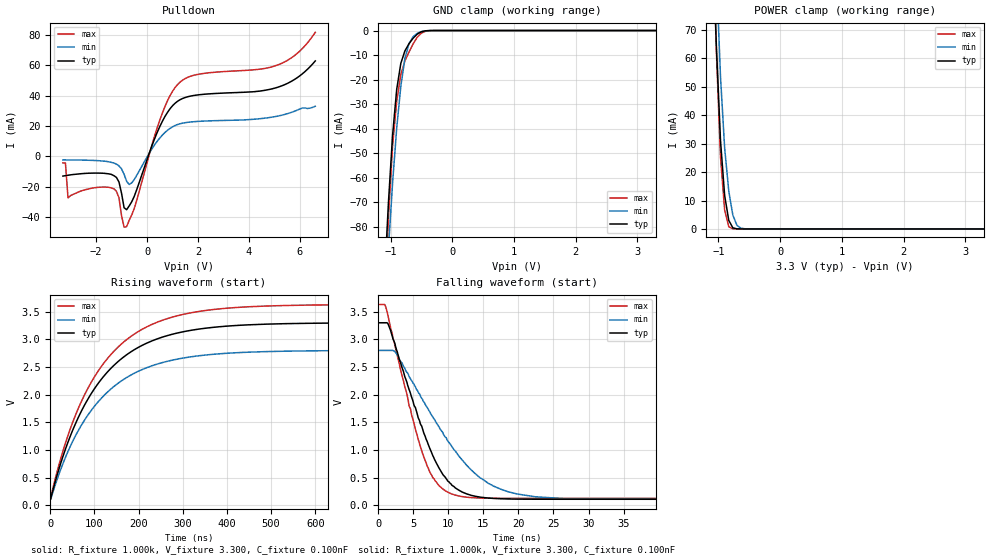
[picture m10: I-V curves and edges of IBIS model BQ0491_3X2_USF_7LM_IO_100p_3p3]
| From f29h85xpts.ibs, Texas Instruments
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|   Model BQ0491_3X2_USF_7LM_IO_100p_3p3
[Model]   BQ0491_3X2_USF_7LM_IO_100p_3p3
Model_type   I/O_open_drain
Polarity   Non-Inverting
Enable   Active-Low
Vinl =   0.800V
Vinh =   2.000V
Vmeas =  1.650V
Cref =   0.100nF
Rref =   1.000k
Vref =   3.300V
|   typ   min   max
C_comp   1.084pF   1.003pF   1.123pF
[Model Spec]
Vinh   2.000V   2.000V   2.000V
Vinl   0.800V   0.800V   0.800V
[Temperature Range]   25   155   -40
[Voltage Range]   3.300V   2.800V   3.630V
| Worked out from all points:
|   slope of the pulldown table from 0 to 0.495 V, typ, clamps not added: 22.9 ohm
|   GND clamp passes 1 mA (typ) near -0.53 V on its own axis
|   POWER clamp passes 1 mA (typ) near -0.78 V on its own axis
|   rising waveform, R_fixture 1.000k, V_fixture 3.300, C_fixture 0.100nF: 20-80 % time 140ns typ, 140ns min, 140ns max; typ from 0.109 V to 3.3 V
|   falling waveform, R_fixture 1.000k, V_fixture 3.300, C_fixture 0.100nF: 20-80 % time 5.42ns typ, 8.49ns min, 4.34ns max; typ from 3.3 V to 0.109 V
[Pulldown]
|Voltage   I(typ)   I(min)   I(max)
-3.3V     -13.02mA   -2.341mA   -4.302mA
-3.2V     -12.73mA   -2.337mA   -4.378mA
-3.1V     -12.44mA   -2.348mA   -27.4mA
-1.3V     -12.73mA   -4.396mA   -21.37mA
-1.1V     -16.92mA   -6.309mA   -27.33mA
-900mV    -33.88mA   -11.82mA   -46.69mA
-800mV    -35.17mA   -16.44mA   -46.34mA
-600mV    -29.93mA   -17.47mA   -38.61mA
500mV     19.62mA    12.09mA    23.89mA
1.2V      36.37mA    21.01mA    47.41mA
5.1V      45.45mA    26.46mA    60.14mA
6.6V      62.95mA    33.05mA    81.82mA
[GND_clamp]
|Voltage   I(typ)   I(min)   I(max)
-3.3V     -1.477A    -1.275A    -1.767A
-1.1V     -102.3mA   -117.4mA   -113.6mA
-1.033V   -69.62mA   -88.44mA   -75.69mA
-967mV    -42.73mA   -62.13mA   -47.02mA
-900mV    -23.96mA   -39.74mA   -28.87mA
-833mV    -13.32mA   -22.64mA   -17.88mA
-767mV    -8.289mA   -11.35mA   -12.33mA
-700mV    -5.352mA   -5.293mA   -8.734mA
-567mV    -1.458mA   -1.135mA   -2.736mA
-433mV    -112.7uA   -134.1uA   -294.8uA
-300mV    -3.58uA    -9.04uA    -6.616uA
3.3V      0A         0A         0A
[POWER_clamp]
|Voltage   I(typ)   I(min)   I(max)
-3.3V     1.901A     2.191A     2.069A
-1.1V     105.6mA    134.8mA    109.4mA
-1.033V   63.91mA    89.93mA    62.06mA
-967mV    31.18mA    53.67mA    25.42mA
-900mV    11.84mA    28.57mA    6.708mA
-833mV    3.029mA    13.38mA    772.2uA
-767mV    401uA      4.887mA    44.81uA
-700mV    39.92uA    1.256mA    4.586uA
-633mV    5.005uA    258uA      1.414uA
-567mV    1.06uA     50.07uA    519.2nA
3.3V      0A         0A         0A
[Ramp]
| variable   typ   min   max
dV/dt_r   1.914/1.296n   1.615/1.263n   2.103/1.336n
dV/dt_f   1.914/0.125n   1.615/0.208n   2.103/98.310p
R_load = 1.000k
[Rising Waveform]
R_fixture= 1.000k
V_fixture= 3.300
V_fixture_min= 2.800
V_fixture_max= 3.630
C_fixture= 0.100nF
|time   V(typ)   V(min)   V(max)
0s        109.4mV    108.1mV    125.7mV
28.1ns    870.1mV    742.6mV    964.8mV
54.1ns    1.421V     1.21V      1.57V
84.3ns    1.907V     1.621V     2.102V
116.3ns   2.286V     1.941V     2.517V
153.3ns   2.597V     2.205V     2.859V
195.3ns   2.837V     2.408V     3.121V
302.3ns   3.14V      2.664V     3.454V
587.3ns   3.29V      2.792V     3.62V
2us       3.3V       2.8V       3.63V
[Falling Waveform]
R_fixture= 1.000k
V_fixture= 3.300
V_fixture_min= 2.800
V_fixture_max= 3.630
C_fixture= 0.100nF
|time   V(typ)   V(min)   V(max)
0s        3.3V       2.8V       3.63V
1.4ns     3.282V     2.8V       3.427V
2.6ns     2.816V     2.741V     2.774V
5.7ns     1.585V     2.045V     1.195V
7.8ns     894.1mV    1.595V     499.1mV
11ns      314.6mV    981.5mV    184.4mV
15.7ns    131.7mV    398.5mV    128.4mV
22.4ns    110mV      154.5mV    125.7mV
48.3ns    109.3mV    108.2mV    125.7mV
2us       109.3mV    108.1mV    125.7mV
